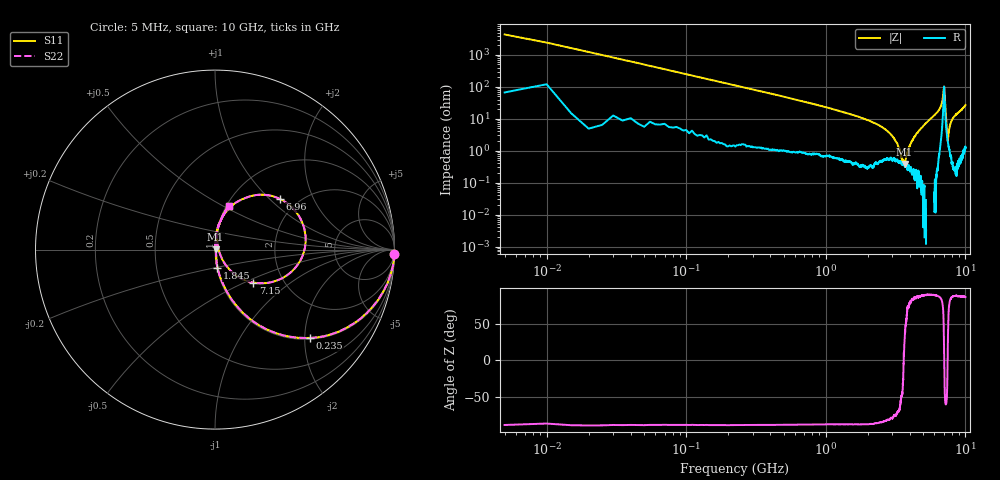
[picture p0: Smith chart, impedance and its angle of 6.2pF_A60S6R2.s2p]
! Amotech Co.,Ltd.
! http://www.amotech.co.kr/
! Part Number: A60S6R2
! These Parameters are Measured in Series Mode Connection
! Operation Temp=25[degC], DC Bias Voltage=0[V]
! Freq. Start=5[MHz] Stop=10[GHz], 2000[Steps]
! Date: Monday, July 13, 2020, 01:31:32
# GHZ S RI R 50.000000
!Freq.(Hz) S11(Real) S11(Imag) S21(Real) S21(Imag) S12(Real) S12(Imag) S22(Real) S22(Imag)
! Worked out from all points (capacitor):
!   2000 points, 5 MHz to 10 GHz, reference 50 ohm
!   read as one part in series: C = 6.41 pF near 55 MHz
!   lowest |Z| = 384 mohm at 3.665 GHz (marker M1)
!   series resonance near 3.615 GHz, so ESL is about 300 pH
!   S11 on the Smith chart (normalised r, x): 5 MHz: 2, -87; 235 MHz: 1.03, -2.12; 1.845 GHz: 1.01, -0.21; 6.96 GHz: 1.62, +1.16; 7.15 GHz: 1.41, -0.56; 10 GHz: 1.03, +0.54
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0.005  0.9991 -0.023  0.000882 0.023  0.000882 0.023  0.9991 -0.023
0.09  0.8796 -0.3165  0.1204 0.3165  0.1204 0.3165  0.8796 -0.3165
0.235  0.5284 -0.4922  0.4716 0.4922  0.4716 0.4922  0.5284 -0.4922
0.41  0.2702 -0.4356  0.7298 0.4356  0.7298 0.4356  0.2702 -0.4356
0.645  0.1293 -0.3235  0.8707 0.3235  0.8707 0.3235  0.1293 -0.3235
1.675  0.0178 -0.1164  0.9822 0.1164  0.9822 0.1164  0.0178 -0.1164
1.845  0.0136 -0.1013  0.9864 0.1013  0.9864 0.1013  0.0136 -0.1013
2.855  0.0066 -0.0352  0.9934 0.0352  0.9934 0.0352  0.0066 -0.0352
3.34  0.00465 -0.0112  0.9954 0.0112  0.9954 0.0112  0.00465 -0.0112
3.54  0.00369 -0.00365  0.9963 0.00365  0.9963 0.00365  0.00369 -0.00365
3.665  0.00336 0.00182  0.9966 -0.00182  0.9966 -0.00182  0.00336 0.00182
4.14  0.00229 0.0198  0.9977 -0.0198  0.9977 -0.0198  0.00229 0.0198
5.005  0.00369 0.0603  0.9963 -0.0603  0.9963 -0.0603  0.00369 0.0603
6.67  0.0739 0.2245  0.9261 -0.2245  0.9261 -0.2245  0.0739 0.2245
6.96  0.3615 0.2819  0.6385 -0.2819  0.6385 -0.2819  0.3615 0.2819
7.045  0.5012 0.0106  0.4988 -0.0106  0.4988 -0.0106  0.5012 0.0106
7.15  0.2121 -0.1835  0.7879 0.1835  0.7879 0.1835  0.2121 -0.1835
7.265  0.0667 -0.0943  0.9333 0.0943  0.9333 0.0943  0.0667 -0.0943
7.475  0.0192 0.00478  0.9808 -0.00478  0.9808 -0.00478  0.0192 0.00478
7.795  0.0113 0.0661  0.9887 -0.0661  0.9887 -0.0661  0.0113 0.0661
8.335  0.0162 0.1166  0.9838 -0.1166  0.9838 -0.1166  0.0162 0.1166
10  0.0778 0.245  0.9222 -0.245  0.9222 -0.245  0.0778 0.245
